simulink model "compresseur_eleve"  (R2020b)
settings: Solver=VariableStepAuto  StartTime=0.0  StopTime=1  RelTol=1e-3
PreLoadFcn:
  | compresseur_7_DataFile
model workspace: external: MATLAB File (data not in the file)
undefined symbols (not defined in the file or in its folder): deg, kg, m, mm, N, s, smiData, X, Y, Z
libraries: sm_lib x91, fl_lib x8, nesl_utility x5, ee_lib x1
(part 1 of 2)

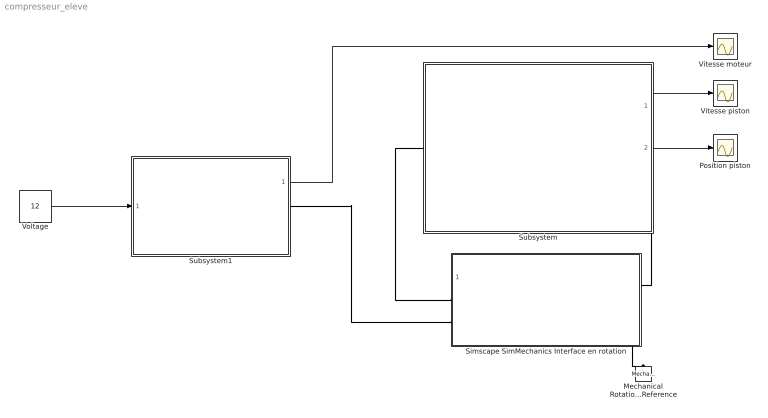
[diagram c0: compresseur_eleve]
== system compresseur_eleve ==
  Mechanical Rotational Reference : fl_lib/Mechanical/Rotational Elements/Mechanical Rotational Reference
  Position piston : Scope
  Simscape SimMechanics Interface en rotation : Subsystem
  Subsystem : Subsystem
  Subsystem1 : Subsystem
  Vitesse moteur : Scope
  Vitesse piston : Scope
  Voltage : Constant  Value=12  VectorParams1D=off  SampleTime=-1
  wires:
  Subsystem/1(output) -> Vitesse piston/1
  Subsystem/2(output1) -> Position piston/1
  Voltage/1 -> Subsystem1/1(input0)
  Subsystem1/1(vitesse de rotation du moteur en tr/mn) -> Vitesse moteur/1
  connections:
  Simscape SimMechanics Interface en rotation/RConn2 -- Mechanical Rotational Reference/LConn1
  Simscape SimMechanics Interface en rotation/LConn1 -- Subsystem/LConn1
  Simscape SimMechanics Interface en rotation/RConn1 -- Subsystem/RConn1
  Simscape SimMechanics Interface en rotation/LConn2 -- Subsystem1/RConn1

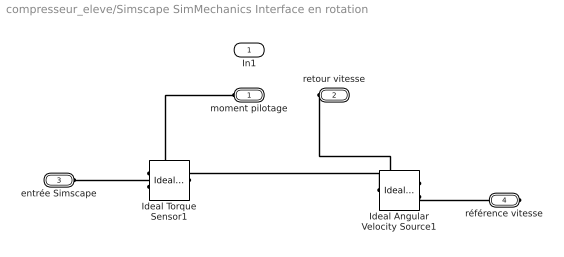
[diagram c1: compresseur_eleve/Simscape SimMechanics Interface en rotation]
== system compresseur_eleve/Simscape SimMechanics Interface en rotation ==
  In1 : Inport
  Ideal Angular Velocity Source1 : fl_lib/Mechanical/Mechanical Sources/Ideal Angular Velocity Source
  Ideal Torque Sensor1 : fl_lib/Mechanical/Mechanical Sensors/Ideal Torque Sensor
  moment pilotage : PMIOPort  Side=Left
  retour vitesse : PMIOPort  Port=2  Side=Right
  entrée Simscape : PMIOPort  Port=3  Side=Left
  référence vitesse : PMIOPort  Port=4  Side=Right
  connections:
  Ideal Angular Velocity Source1/RConn2 -- référence vitesse/RConn1
  Ideal Torque Sensor1/RConn2 -- moment pilotage/RConn1
  Ideal Angular Velocity Source1/LConn1 -- Ideal Torque Sensor1/RConn1
  Ideal Torque Sensor1/LConn1 -- entrée Simscape/RConn1
  retour vitesse/RConn1 -- Ideal Angular Velocity Source1/RConn1

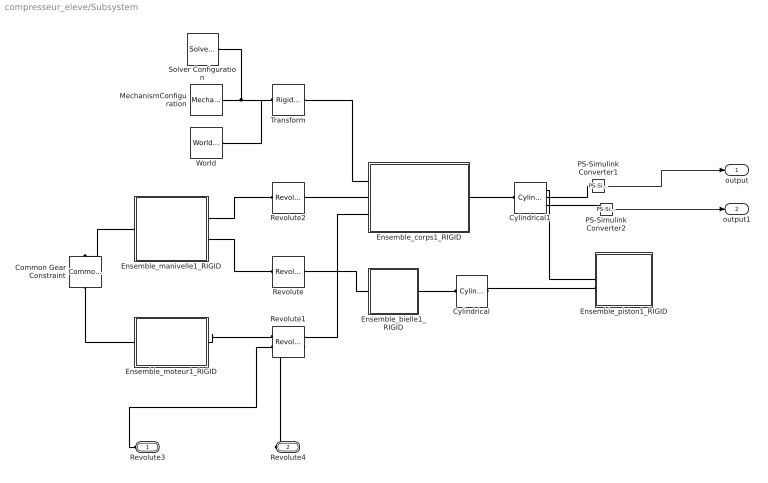
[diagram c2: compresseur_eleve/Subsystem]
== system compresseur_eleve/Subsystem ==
  Common Gear Constraint : sm_lib/Gears and Couplings/Gears/Common Gear Constraint  GearType=External  SpecificationType=CenterDistanceRatio  CenterDistance=22.5  CenterDistanceUnits=mm  GearRatio=3  BaseGearRadius=10.0  BaseGearRadiusUnits=cm  FollGearRadius=10.0  FollGearRadiusUnits=cm  AssemblyGearRotation=Free
  Cylindrical : sm_lib/Joints/Cylindrical Joint  JointMode=Normal  SenseConstraintForce=off  SenseConstraintForceX=off  SenseConstraintForceY=off  SenseConstraintForceZ=off  SenseConstraintTorque=off  SenseConstraintTorqueX=off  SenseConstraintTorqueY=off  SenseConstraintTorqueZ=off  SenseTotalForce=off  SenseTotalForceX=off  SenseTotalForceY=off  SenseTotalForceZ=off  SenseTotalTorque=off  SenseTotalTorqueX=off  SenseTotalTorqueY=off  SenseTotalTorqueZ=off  CompositeWrenchDir=FollowerOnBase  CompositeWrenchFrame=BaseFrame  PzEquilibriumPosition=0  PzEquilibriumPositionUnits=m  PzSpringStiffness=0  PzSpringStiffnessUnits=N/m  PzDampingCoefficient=0  PzDampingCoefficientUnits=N/(m/s)  PzTorqueActuationMode=NoTorque  PzMotionActuationMode=ComputedMotion  PzSensePosition=off  PzSenseVelocity=off  PzSenseAcceleration=off  PzSenseTorqueForce=off  PzSenseLowerLimitTorqueForce=off  PzSenseUpperLimitTorqueForce=off  PzLowerLimitSpecify=off  PzLowerLimitBound=-1  PzLowerLimitBoundUnits=m  PzLowerLimitStiffness=1e6  PzLowerLimitStiffnessUnits=N/m  PzLowerLimitDamping=1e3  PzLowerLimitDampingUnits=N/(m/s)  PzLowerLimitTransitionRegionWidth=1e-4  PzLowerLimitTransitionRegionWidthUnits=m  PzUpperLimitSpecify=off  PzUpperLimitBound=1  PzUpperLimitBoundUnits=m  PzUpperLimitStiffness=1e6  PzUpperLimitStiffnessUnits=N/m  PzUpperLimitDamping=1e3  PzUpperLimitDampingUnits=N/(m/s)  PzUpperLimitTransitionRegionWidth=1e-4  PzUpperLimitTransitionRegionWidthUnits=m  PzPositionTargetSpecify=off  PzPositionTargetPriority=High  PzPositionTargetValue=0  PzPositionTargetValueUnits=m  PzVelocityTargetSpecify=off  PzVelocityTargetPriority=High  PzVelocityTargetValue=0  PzVelocityTargetValueUnits=m/s  RzEquilibriumPosition=0  RzEquilibriumPositionUnits=deg  RzSpringStiffness=0  RzSpringStiffnessUnits=N*m/deg  RzDampingCoefficient=0  RzDampingCoefficientUnits=N*m/(deg/s)  RzTorqueActuationMode=NoTorque  RzMotionActuationMode=ComputedMotion  RzSensePosition=off  RzSenseVelocity=off  RzSenseAcceleration=off  RzSenseTorqueForce=off  RzSenseLowerLimitTorqueForce=off  RzSenseUpperLimitTorqueForce=off  RzLowerLimitSpecify=off  RzLowerLimitBound=-90  RzLowerLimitBoundUnits=deg  RzLowerLimitStiffness=1e4  RzLowerLimitStiffnessUnits=N*m/deg  RzLowerLimitDamping=10  RzLowerLimitDampingUnits=N*m/(deg/s)  RzLowerLimitTransitionRegionWidth=0.1  RzLowerLimitTransitionRegionWidthUnits=deg  RzUpperLimitSpecify=off  RzUpperLimitBound=90  RzUpperLimitBoundUnits=deg  RzUpperLimitStiffness=1e4  RzUpperLimitStiffnessUnits=N*m/deg  RzUpperLimitDamping=10  RzUpperLimitDampingUnits=N*m/(deg/s)  RzUpperLimitTransitionRegionWidth=0.1  RzUpperLimitTransitionRegionWidthUnits=deg  RzPositionTargetSpecify=off  RzPositionTargetPriority=High  RzPositionTargetValue=0  RzPositionTargetValueUnits=deg  RzVelocityTargetSpecify=off  RzVelocityTargetPriority=High  RzVelocityTargetValue=0  RzVelocityTargetValueUnits=deg/s
  Cylindrical1 : sm_lib/Joints/Cylindrical Joint  JointMode=Normal  SenseConstraintForce=off  SenseConstraintForceX=off  SenseConstraintForceY=off  SenseConstraintForceZ=off  SenseConstraintTorque=off  SenseConstraintTorqueX=off  SenseConstraintTorqueY=off  SenseConstraintTorqueZ=off  SenseTotalForce=off  SenseTotalForceX=off  SenseTotalForceY=off  SenseTotalForceZ=off  SenseTotalTorque=off  SenseTotalTorqueX=off  SenseTotalTorqueY=off  SenseTotalTorqueZ=off  CompositeWrenchDir=FollowerOnBase  CompositeWrenchFrame=BaseFrame  PzEquilibriumPosition=0  PzEquilibriumPositionUnits=m  PzSpringStiffness=0  PzSpringStiffnessUnits=N/m  PzDampingCoefficient=0  PzDampingCoefficientUnits=N/(m/s)  PzTorqueActuationMode=NoTorque  PzMotionActuationMode=ComputedMotion  PzSensePosition=on  PzSenseVelocity=on  PzSenseAcceleration=off  PzSenseTorqueForce=off  PzSenseLowerLimitTorqueForce=off  PzSenseUpperLimitTorqueForce=off  PzLowerLimitSpecify=off  PzLowerLimitBound=-1  PzLowerLimitBoundUnits=m  PzLowerLimitStiffness=1e6  PzLowerLimitStiffnessUnits=N/m  PzLowerLimitDamping=1e3  PzLowerLimitDampingUnits=N/(m/s)  PzLowerLimitTransitionRegionWidth=1e-4  PzLowerLimitTransitionRegionWidthUnits=m  PzUpperLimitSpecify=off  PzUpperLimitBound=1  PzUpperLimitBoundUnits=m  PzUpperLimitStiffness=1e6  PzUpperLimitStiffnessUnits=N/m  PzUpperLimitDamping=1e3  PzUpperLimitDampingUnits=N/(m/s)  PzUpperLimitTransitionRegionWidth=1e-4  PzUpperLimitTransitionRegionWidthUnits=m  PzPositionTargetSpecify=on  PzPositionTargetPriority=Low  PzPositionTargetValue=smiData.CylindricalJoint(2).Pz.Pos  PzPositionTargetValueUnits=mm  PzVelocityTargetSpecify=off  PzVelocityTargetPriority=High  PzVelocityTargetValue=0  PzVelocityTargetValueUnits=m/s  RzEquilibriumPosition=0  RzEquilibriumPositionUnits=deg  RzSpringStiffness=0  RzSpringStiffnessUnits=N*m/deg  RzDampingCoefficient=0  RzDampingCoefficientUnits=N*m/(deg/s)  RzTorqueActuationMode=NoTorque  RzMotionActuationMode=ComputedMotion  RzSensePosition=off  RzSenseVelocity=off  RzSenseAcceleration=off  RzSenseTorqueForce=off  RzSenseLowerLimitTorqueForce=off  RzSenseUpperLimitTorqueForce=off  RzLowerLimitSpecify=off  RzLowerLimitBound=-90  RzLowerLimitBoundUnits=deg  RzLowerLimitStiffness=1e4  RzLowerLimitStiffnessUnits=N*m/deg  RzLowerLimitDamping=10  RzLowerLimitDampingUnits=N*m/(deg/s)  RzLowerLimitTransitionRegionWidth=0.1  RzLowerLimitTransitionRegionWidthUnits=deg  RzUpperLimitSpecify=off  RzUpperLimitBound=90  RzUpperLimitBoundUnits=deg  RzUpperLimitStiffness=1e4  RzUpperLimitStiffnessUnits=N*m/deg  RzUpperLimitDamping=10  RzUpperLimitDampingUnits=N*m/(deg/s)  RzUpperLimitTransitionRegionWidth=0.1  RzUpperLimitTransitionRegionWidthUnits=deg  RzPositionTargetSpecify=on  RzPositionTargetPriority=Low  RzPositionTargetValue=smiData.CylindricalJoint(2).Rz.Pos  RzPositionTargetValueUnits=deg  RzVelocityTargetSpecify=off  RzVelocityTargetPriority=High  RzVelocityTargetValue=0  RzVelocityTargetValueUnits=deg/s
  Ensemble_bielle1_RIGID : Subsystem
  Ensemble_corps1_RIGID : Subsystem
  Ensemble_manivelle1_RIGID : Subsystem
  Ensemble_moteur1_RIGID : Subsystem
  Ensemble_piston1_RIGID : Subsystem
  MechanismConfiguration : sm_lib/Utilities/Mechanism Configuration  UniformGravity=Constant  GravityVector=[0 -9.80665 0]  GravityVectorUnits=m/s^2  GravityUnits=m/s^2  LinearizationDelta=0.001  JointModeTransitionNonlinearIterations=2
  PS-Simulink Converter1 : nesl_utility/PS-Simulink Converter  PhysicalDomain=network_engine_domain  SubClassName=ps_output  LeftPortType=input  RightPortType=output  PseudoPeriodic=off  Frequencies=[]  Unit=inherit  AffineConversion=off
  PS-Simulink Converter2 : nesl_utility/PS-Simulink Converter  PhysicalDomain=network_engine_domain  SubClassName=ps_output  LeftPortType=input  RightPortType=output  PseudoPeriodic=off  Frequencies=[]  Unit=inherit  AffineConversion=off
  Revolute : sm_lib/Joints/Revolute Joint  JointMode=Normal  SenseConstraintForce=off  SenseConstraintForceX=off  SenseConstraintForceY=off  SenseConstraintForceZ=off  SenseConstraintTorque=off  SenseConstraintTorqueX=off  SenseConstraintTorqueY=off  SenseConstraintTorqueZ=off  SenseTotalForce=off  SenseTotalForceX=off  SenseTotalForceY=off  SenseTotalForceZ=off  SenseTotalTorque=off  SenseTotalTorqueX=off  SenseTotalTorqueY=off  SenseTotalTorqueZ=off  CompositeWrenchDir=FollowerOnBase  CompositeWrenchFrame=BaseFrame  EquilibriumPosition=0  EquilibriumPositionUnits=deg  SpringStiffness=0  SpringStiffnessUnits=N*m/deg  DampingCoefficient=0  DampingCoefficientUnits=N*m/(deg/s)  TorqueActuationMode=NoTorque  MotionActuationMode=ComputedMotion  SensePosition=off  SenseVelocity=off  SenseAcceleration=off  SenseTorqueForce=off  SenseLowerLimitTorqueForce=off  SenseUpperLimitTorqueForce=off  LowerLimitSpecify=off  LowerLimitBound=-90  LowerLimitBoundUnits=deg  LowerLimitStiffness=1e4  LowerLimitStiffnessUnits=N*m/deg  LowerLimitDamping=10  LowerLimitDampingUnits=N*m/(deg/s)  LowerLimitTransitionRegionWidth=0.1  LowerLimitTransitionRegionWidthUnits=deg  UpperLimitSpecify=off  UpperLimitBound=90  UpperLimitBoundUnits=deg  UpperLimitStiffness=1e4  UpperLimitStiffnessUnits=N*m/deg  UpperLimitDamping=10  UpperLimitDampingUnits=N*m/(deg/s)  UpperLimitTransitionRegionWidth=0.1  UpperLimitTransitionRegionWidthUnits=deg  PositionTargetSpecify=on  PositionTargetPriority=Low  PositionTargetValue=smiData.RevoluteJoint(1).Rz.Pos  PositionTargetValueUnits=deg  VelocityTargetSpecify=off  VelocityTargetPriority=High  VelocityTargetValue=0  VelocityTargetValueUnits=deg/s
  Revolute1 : sm_lib/Joints/Revolute Joint  JointMode=Normal  SenseConstraintForce=off  SenseConstraintForceX=off  SenseConstraintForceY=off  SenseConstraintForceZ=off  SenseConstraintTorque=off  SenseConstraintTorqueX=off  SenseConstraintTorqueY=off  SenseConstraintTorqueZ=off  SenseTotalForce=off  SenseTotalForceX=off  SenseTotalForceY=off  SenseTotalForceZ=off  SenseTotalTorque=off  SenseTotalTorqueX=off  SenseTotalTorqueY=off  SenseTotalTorqueZ=off  CompositeWrenchDir=FollowerOnBase  CompositeWrenchFrame=BaseFrame  EquilibriumPosition=0  EquilibriumPositionUnits=deg  SpringStiffness=0  SpringStiffnessUnits=N*m/deg  DampingCoefficient=0  DampingCoefficientUnits=N*m/(deg/s)  TorqueActuationMode=InputTorque  MotionActuationMode=ComputedMotion  SensePosition=off  SenseVelocity=on  SenseAcceleration=off  SenseTorqueForce=off  SenseLowerLimitTorqueForce=off  SenseUpperLimitTorqueForce=off  LowerLimitSpecify=off  LowerLimitBound=-90  LowerLimitBoundUnits=deg  LowerLimitStiffness=1e4  LowerLimitStiffnessUnits=N*m/deg  LowerLimitDamping=10  LowerLimitDampingUnits=N*m/(deg/s)  LowerLimitTransitionRegionWidth=0.1  LowerLimitTransitionRegionWidthUnits=deg  UpperLimitSpecify=off  UpperLimitBound=90  UpperLimitBoundUnits=deg  UpperLimitStiffness=1e4  UpperLimitStiffnessUnits=N*m/deg  UpperLimitDamping=10  UpperLimitDampingUnits=N*m/(deg/s)  UpperLimitTransitionRegionWidth=0.1  UpperLimitTransitionRegionWidthUnits=deg  PositionTargetSpecify=on  PositionTargetPriority=Low  PositionTargetValue=smiData.RevoluteJoint(2).Rz.Pos  PositionTargetValueUnits=deg  VelocityTargetSpecify=off  VelocityTargetPriority=High  VelocityTargetValue=0  VelocityTargetValueUnits=deg/s
  Revolute2 : sm_lib/Joints/Revolute Joint  JointMode=Normal  SenseConstraintForce=off  SenseConstraintForceX=off  SenseConstraintForceY=off  SenseConstraintForceZ=off  SenseConstraintTorque=off  SenseConstraintTorqueX=off  SenseConstraintTorqueY=off  SenseConstraintTorqueZ=off  SenseTotalForce=off  SenseTotalForceX=off  SenseTotalForceY=off  SenseTotalForceZ=off  SenseTotalTorque=off  SenseTotalTorqueX=off  SenseTotalTorqueY=off  SenseTotalTorqueZ=off  CompositeWrenchDir=FollowerOnBase  CompositeWrenchFrame=BaseFrame  EquilibriumPosition=0  EquilibriumPositionUnits=deg  SpringStiffness=0  SpringStiffnessUnits=N*m/deg  DampingCoefficient=0  DampingCoefficientUnits=N*m/(deg/s)  TorqueActuationMode=NoTorque  MotionActuationMode=ComputedMotion  SensePosition=off  SenseVelocity=off  SenseAcceleration=off  SenseTorqueForce=off  SenseLowerLimitTorqueForce=off  SenseUpperLimitTorqueForce=off  LowerLimitSpecify=off  LowerLimitBound=-90  LowerLimitBoundUnits=deg  LowerLimitStiffness=1e4  LowerLimitStiffnessUnits=N*m/deg  LowerLimitDamping=10  LowerLimitDampingUnits=N*m/(deg/s)  LowerLimitTransitionRegionWidth=0.1  LowerLimitTransitionRegionWidthUnits=deg  UpperLimitSpecify=off  UpperLimitBound=90  UpperLimitBoundUnits=deg  UpperLimitStiffness=1e4  UpperLimitStiffnessUnits=N*m/deg  UpperLimitDamping=10  UpperLimitDampingUnits=N*m/(deg/s)  UpperLimitTransitionRegionWidth=0.1  UpperLimitTransitionRegionWidthUnits=deg  PositionTargetSpecify=on  PositionTargetPriority=Low  PositionTargetValue=smiData.RevoluteJoint(3).Rz.Pos  PositionTargetValueUnits=deg  VelocityTargetSpecify=off  VelocityTargetPriority=High  VelocityTargetValue=0  VelocityTargetValueUnits=deg/s
  Solver Configuration : nesl_utility/Solver Configuration  PhysicalDomain=network_engine_domain  SubClassName=solver  LeftPortType=input  RightPortType=generic  Tones=[]  Harmonics=[]  SimulateNoise=off  Profile=off  UseLocalSampling=off  EnableSwitchedLinearOptims=on  FrequencyDomain=off  UseCCode=off  RelTol=0.001  AbsTol=1e-06  MinStep=1e-09  ToWorkspace=off  RevertToSquareIcSolve=off  NumHomotopyIterations=100  PhasorMode=off  PhasorModeNumHarmonics=1  DoDC=off  ResidualTolerance=1e-09  UseLocalSolver=off  LocalSolverChoice=NE_BACKWARD_EULER_ADVANCER  LocalSolverSampleTime=0.001  DoFixedCost=off  MaxNonlinIter=3  MaxModeIter=2  ComputeImpulses=off  ImpulseIterations=2  LinearAlgebra=auto  EquationFormulation=NE_TIME_EF  DelaysMemoryBudget=1024  AutomaticFiltering=on  FilteringTimeConstant=0.001  PartitionStorageMethod=AS_NEEDED  PartitionMemoryBudget=1024  PartitionMethod=ROBUST
  Transform : sm_lib/Frames and Transforms/Rigid Transform  TranslationMethod=Cartesian  TranslationStandardOffset=0  TranslationLengthUnit=mm  TranslationStandardAxis=+Z  TranslationCartesianOffset=smiData.RigidTransform(33).translation  TranslationROffset=0  TranslationROffsetUnits=m  TranslationZOffset=0  TranslationZOffsetUnits=m  TranslationThetaOffset=0  TranslationThetaOffsetUnits=deg  RotationMethod=ArbitraryAxis  RotationAngleUnits=rad  RotationStandardAxis=+Z  RotationAngle=smiData.RigidTransform(33).angle  RotationArbitraryAxis=smiData.RigidTransform(33).axis  FollAlignAxisA=+X  BaseAlignAxisA=+Y  FollAlignAxisB=+Y  BaseAlignAxisB=+Z  RotationSequenceAxes=FollowerAxes  RotationSequence=XYX  RotationSequenceAngles=[0 0 0]  RotationSequenceAnglesUnits=deg  RotationMatrix=[1 0 0; 0 1 0; 0 0 1]
  World : sm_lib/Frames and Transforms/World Frame
  Revolute3 : PMIOPort  Side=Left
  Revolute4 : PMIOPort  Port=2  Side=Right
  output : Outport
  output1 : Outport  Port=2
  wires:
  PS-Simulink Converter2/1 -> output1/1
  PS-Simulink Converter1/1 -> output/1
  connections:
  Transform/LConn1 -- MechanismConfiguration/RConn1 -- Solver Configuration/RConn1 -- World/RConn1
  Cylindrical1/LConn1 -- Ensemble_corps1_RIGID/RConn1
  Ensemble_corps1_RIGID/LConn1 -- Transform/RConn1
  PS-Simulink Converter1/LConn1 -- Cylindrical1/RConn2
  Ensemble_corps1_RIGID/LConn3 -- Revolute1/RConn1
  Ensemble_manivelle1_RIGID/RConn1 -- Revolute2/LConn1
  PS-Simulink Converter2/LConn1 -- Cylindrical1/RConn3
  Revolute3/RConn1 -- Revolute1/LConn2
  Common Gear Constraint/LConn1 -- Ensemble_moteur1_RIGID/LConn1
  Ensemble_manivelle1_RIGID/RConn2 -- Revolute/LConn1
  Cylindrical/RConn1 -- Ensemble_piston1_RIGID/LConn2
  Ensemble_corps1_RIGID/LConn2 -- Revolute2/RConn1
  Cylindrical1/RConn1 -- Ensemble_piston1_RIGID/LConn1
  Cylindrical/LConn1 -- Ensemble_bielle1_RIGID/RConn1
  Ensemble_moteur1_RIGID/RConn1 -- Revolute1/LConn1
  Ensemble_manivelle1_RIGID/LConn1 -- Common Gear Constraint/RConn1
  Ensemble_bielle1_RIGID/LConn1 -- Revolute/RConn1
  Revolute4/RConn1 -- Revolute1/RConn2

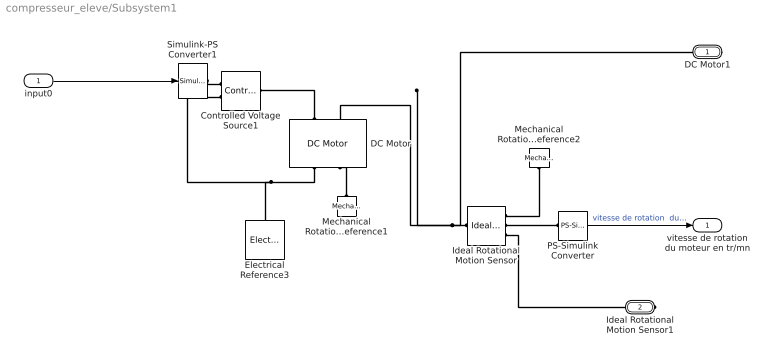
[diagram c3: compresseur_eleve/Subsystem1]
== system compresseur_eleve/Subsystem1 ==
  input0 : Inport
  Controlled Voltage Source1 : fl_lib/Electrical/Electrical Sources/Controlled Voltage Source
  DC Motor : ee_lib/Electromechanical/Brushed Motors/DC Motor  field_option=ee.enum.field_option.pm  Rf=100 Ohm  Lf=1 H  Laf=0.15 H  If0=0 A  parameterization=1  Ra=3.9 Ohm  La=0.1 mH  emf_or_torque=2  Kv=7.2e-6 V/rpm  Ki=1e-2 N*m/A  T_stall=2.4e-4 N*m  w_max=1.91e+4 rpm  w_rated=1.5e+4 rpm  P_rated=0.08 W  V_rated=1.5 V  J=80 g*cm^2  lam_param=1  lam=0 N*m/(rad/s)  i_noload=0 A  V_i_noload=1.5 V  speed0=0 rpm  enable_fault_armature=ee.enum.faults.faultEnable.no  rev_faulted=1 / 3  G_faulted_armature=1e-5 S  fault_trigger_armature=ee.enum.faults.faultTrigger.temporal  t_fault_armature=1 s  max_permissible_current_armature=inf A  t_fail_on_current_armature=1 s  enable_fault_field=ee.enum.faults.faultEnable.no  G_faulted_field=1e-5 S  fault_trigger_field=ee.enum.faults.faultTrigger.temporal  t_fault_field=1 s  max_permissible_current_field=inf A  t_fail_on_current_field=1 s  fault_action=ee.enum.faults.faultAction.none  alpha=3.93e-3 1/K  Tmeas=25 degC  thermal_mass=100 J/K  initial_temperature=25 degC
  Electrical Reference3 : fl_lib/Electrical/Electrical Elements/Electrical Reference
  Ideal Rotational Motion Sensor : fl_lib/Mechanical/Mechanical Sensors/Ideal Rotational Motion Sensor  wrap_angle=simscape.enum.onoff.off  offset=0 rad
  Mechanical Rotational Reference1 : fl_lib/Mechanical/Rotational Elements/Mechanical Rotational Reference
  Mechanical Rotational Reference2 : fl_lib/Mechanical/Rotational Elements/Mechanical Rotational Reference
  PS-Simulink Converter : nesl_utility/PS-Simulink Converter  PhysicalDomain=network_engine_domain  SubClassName=ps_output  LeftPortType=input  RightPortType=output  PseudoPeriodic=off  Frequencies=[]  Unit=rpm  AffineConversion=off
  Simulink-PS Converter1 : nesl_utility/Simulink-PS Converter  PhysicalDomain=network_engine_domain  SubClassName=ps_input  LeftPortType=input  RightPortType=output  PseudoPeriodic=off  Frequencies=[]  NoiseDistribution=none  NoiseParameters=[]  Unit=V  AffineConversion=off  FilteringAndDerivatives=zero  SimscapeFilterOrder=1  InputFilterTimeConstant=0.001  UdotUserProvided=1
  DC Motor1 : PMIOPort  Side=Right
  Ideal Rotational Motion Sensor1 : PMIOPort  Port=2  Side=Right
  vitesse de rotation du moteur en tr/mn : Outport
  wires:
  input0/1 -> Simulink-PS Converter1/1
  PS-Simulink Converter/1 -> vitesse de rotation du moteur en tr/mn/1  "vitesse de rotation  du moteur en tr/mn"
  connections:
  Mechanical Rotational Reference2/LConn1 -- Ideal Rotational Motion Sensor/RConn1
  DC Motor/RConn1 -- Controlled Voltage Source1/RConn2 -- Electrical Reference3/LConn1
  Ideal Rotational Motion Sensor/RConn2 -- PS-Simulink Converter/LConn1
  Ideal Rotational Motion Sensor/LConn1 -- DC Motor1/RConn1 -- DC Motor/LConn2
  DC Motor/LConn1 -- Controlled Voltage Source1/LConn1
  Ideal Rotational Motion Sensor/RConn3 -- Ideal Rotational Motion Sensor1/RConn1
  Simulink-PS Converter1/RConn1 -- Controlled Voltage Source1/RConn1
  Mechanical Rotational Reference1/LConn1 -- DC Motor/RConn2

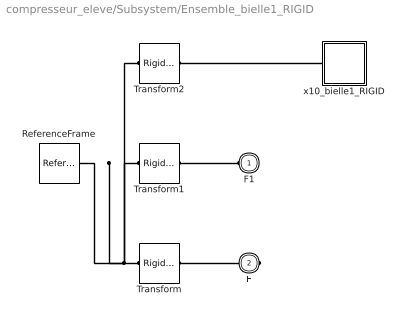
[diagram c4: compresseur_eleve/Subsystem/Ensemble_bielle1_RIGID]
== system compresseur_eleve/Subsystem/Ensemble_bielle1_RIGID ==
  ReferenceFrame : sm_lib/Frames and Transforms/Reference Frame
  Transform : sm_lib/Frames and Transforms/Rigid Transform  TranslationMethod=Cartesian  TranslationStandardOffset=0  TranslationLengthUnit=mm  TranslationStandardAxis=+Z  TranslationCartesianOffset=smiData.RigidTransform(1).translation  TranslationROffset=0  TranslationROffsetUnits=m  TranslationZOffset=0  TranslationZOffsetUnits=m  TranslationThetaOffset=0  TranslationThetaOffsetUnits=deg  RotationMethod=ArbitraryAxis  RotationAngleUnits=rad  RotationStandardAxis=+Z  RotationAngle=smiData.RigidTransform(1).angle  RotationArbitraryAxis=smiData.RigidTransform(1).axis  FollAlignAxisA=+X  BaseAlignAxisA=+Y  FollAlignAxisB=+Y  BaseAlignAxisB=+Z  RotationSequenceAxes=FollowerAxes  RotationSequence=XYX  RotationSequenceAngles=[0 0 0]  RotationSequenceAnglesUnits=deg  RotationMatrix=[1 0 0; 0 1 0; 0 0 1]
  Transform1 : sm_lib/Frames and Transforms/Rigid Transform  TranslationMethod=Cartesian  TranslationStandardOffset=0  TranslationLengthUnit=mm  TranslationStandardAxis=+Z  TranslationCartesianOffset=smiData.RigidTransform(4).translation  TranslationROffset=0  TranslationROffsetUnits=m  TranslationZOffset=0  TranslationZOffsetUnits=m  TranslationThetaOffset=0  TranslationThetaOffsetUnits=deg  RotationMethod=ArbitraryAxis  RotationAngleUnits=rad  RotationStandardAxis=+Z  RotationAngle=smiData.RigidTransform(4).angle  RotationArbitraryAxis=smiData.RigidTransform(4).axis  FollAlignAxisA=+X  BaseAlignAxisA=+Y  FollAlignAxisB=+Y  BaseAlignAxisB=+Z  RotationSequenceAxes=FollowerAxes  RotationSequence=XYX  RotationSequenceAngles=[0 0 0]  RotationSequenceAnglesUnits=deg  RotationMatrix=[1 0 0; 0 1 0; 0 0 1]
  Transform2 : sm_lib/Frames and Transforms/Rigid Transform  TranslationMethod=Cartesian  TranslationStandardOffset=0  TranslationLengthUnit=mm  TranslationStandardAxis=+Z  TranslationCartesianOffset=smiData.RigidTransform(20).translation  TranslationROffset=0  TranslationROffsetUnits=m  TranslationZOffset=0  TranslationZOffsetUnits=m  TranslationThetaOffset=0  TranslationThetaOffsetUnits=deg  RotationMethod=ArbitraryAxis  RotationAngleUnits=rad  RotationStandardAxis=+Z  RotationAngle=smiData.RigidTransform(20).angle  RotationArbitraryAxis=smiData.RigidTransform(20).axis  FollAlignAxisA=+X  BaseAlignAxisA=+Y  FollAlignAxisB=+Y  BaseAlignAxisB=+Z  RotationSequenceAxes=FollowerAxes  RotationSequence=XYX  RotationSequenceAngles=[0 0 0]  RotationSequenceAnglesUnits=deg  RotationMatrix=[1 0 0; 0 1 0; 0 0 1]
  x10_bielle1_RIGID : Subsystem
  F1 : PMIOPort  Side=Left
  F : PMIOPort  Port=2  Side=Right
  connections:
  Transform/LConn1 -- ReferenceFrame/RConn1 -- Transform1/LConn1 -- Transform2/LConn1
  Transform/RConn1 -- F/RConn1
  Transform1/RConn1 -- F1/RConn1
  Transform2/RConn1 -- x10_bielle1_RIGID/LConn1

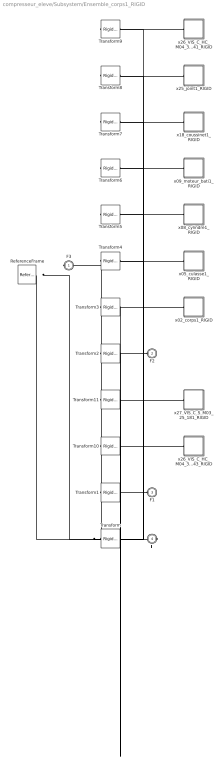
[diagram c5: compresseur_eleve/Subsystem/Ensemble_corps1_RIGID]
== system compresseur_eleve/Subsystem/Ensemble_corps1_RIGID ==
  ReferenceFrame : sm_lib/Frames and Transforms/Reference Frame
  Transform : sm_lib/Frames and Transforms/Rigid Transform  TranslationMethod=Cartesian  TranslationStandardOffset=0  TranslationLengthUnit=mm  TranslationStandardAxis=+Z  TranslationCartesianOffset=smiData.RigidTransform(5).translation  TranslationROffset=0  TranslationROffsetUnits=m  TranslationZOffset=0  TranslationZOffsetUnits=m  TranslationThetaOffset=0  TranslationThetaOffsetUnits=deg  RotationMethod=ArbitraryAxis  RotationAngleUnits=rad  RotationStandardAxis=+Z  RotationAngle=smiData.RigidTransform(5).angle  RotationArbitraryAxis=smiData.RigidTransform(5).axis  FollAlignAxisA=+X  BaseAlignAxisA=+Y  FollAlignAxisB=+Y  BaseAlignAxisB=+Z  RotationSequenceAxes=FollowerAxes  RotationSequence=XYX  RotationSequenceAngles=[0 0 0]  RotationSequenceAnglesUnits=deg  RotationMatrix=[1 0 0; 0 1 0; 0 0 1]
  Transform1 : sm_lib/Frames and Transforms/Rigid Transform  TranslationMethod=Cartesian  TranslationStandardOffset=0  TranslationLengthUnit=mm  TranslationStandardAxis=+Z  TranslationCartesianOffset=smiData.RigidTransform(8).translation  TranslationROffset=0  TranslationROffsetUnits=m  TranslationZOffset=0  TranslationZOffsetUnits=m  TranslationThetaOffset=0  TranslationThetaOffsetUnits=deg  RotationMethod=ArbitraryAxis  RotationAngleUnits=rad  RotationStandardAxis=+Z  RotationAngle=smiData.RigidTransform(8).angle  RotationArbitraryAxis=smiData.RigidTransform(8).axis  FollAlignAxisA=+X  BaseAlignAxisA=+Y  FollAlignAxisB=+Y  BaseAlignAxisB=+Z  RotationSequenceAxes=FollowerAxes  RotationSequence=XYX  RotationSequenceAngles=[0 0 0]  RotationSequenceAnglesUnits=deg  RotationMatrix=[1 0 0; 0 1 0; 0 0 1]
  Transform10 : sm_lib/Frames and Transforms/Rigid Transform  TranslationMethod=Cartesian  TranslationStandardOffset=0  TranslationLengthUnit=mm  TranslationStandardAxis=+Z  TranslationCartesianOffset=smiData.RigidTransform(18).translation  TranslationROffset=0  TranslationROffsetUnits=m  TranslationZOffset=0  TranslationZOffsetUnits=m  TranslationThetaOffset=0  TranslationThetaOffsetUnits=deg  RotationMethod=ArbitraryAxis  RotationAngleUnits=rad  RotationStandardAxis=+Z  RotationAngle=smiData.RigidTransform(18).angle  RotationArbitraryAxis=smiData.RigidTransform(18).axis  FollAlignAxisA=+X  BaseAlignAxisA=+Y  FollAlignAxisB=+Y  BaseAlignAxisB=+Z  RotationSequenceAxes=FollowerAxes  RotationSequence=XYX  RotationSequenceAngles=[0 0 0]  RotationSequenceAnglesUnits=deg  RotationMatrix=[1 0 0; 0 1 0; 0 0 1]
  Transform11 : sm_lib/Frames and Transforms/Rigid Transform  TranslationMethod=Cartesian  TranslationStandardOffset=0  TranslationLengthUnit=mm  TranslationStandardAxis=+Z  TranslationCartesianOffset=smiData.RigidTransform(19).translation  TranslationROffset=0  TranslationROffsetUnits=m  TranslationZOffset=0  TranslationZOffsetUnits=m  TranslationThetaOffset=0  TranslationThetaOffsetUnits=deg  RotationMethod=ArbitraryAxis  RotationAngleUnits=rad  RotationStandardAxis=+Z  RotationAngle=smiData.RigidTransform(19).angle  RotationArbitraryAxis=smiData.RigidTransform(19).axis  FollAlignAxisA=+X  BaseAlignAxisA=+Y  FollAlignAxisB=+Y  BaseAlignAxisB=+Z  RotationSequenceAxes=FollowerAxes  RotationSequence=XYX  RotationSequenceAngles=[0 0 0]  RotationSequenceAnglesUnits=deg  RotationMatrix=[1 0 0; 0 1 0; 0 0 1]
  Transform2 : sm_lib/Frames and Transforms/Rigid Transform  TranslationMethod=Cartesian  TranslationStandardOffset=0  TranslationLengthUnit=mm  TranslationStandardAxis=+Z  TranslationCartesianOffset=smiData.RigidTransform(10).translation  TranslationROffset=0  TranslationROffsetUnits=m  TranslationZOffset=0  TranslationZOffsetUnits=m  TranslationThetaOffset=0  TranslationThetaOffsetUnits=deg  RotationMethod=ArbitraryAxis  RotationAngleUnits=rad  RotationStandardAxis=+Z  RotationAngle=smiData.RigidTransform(10).angle  RotationArbitraryAxis=smiData.RigidTransform(10).axis  FollAlignAxisA=+X  BaseAlignAxisA=+Y  FollAlignAxisB=+Y  BaseAlignAxisB=+Z  RotationSequenceAxes=FollowerAxes  RotationSequence=XYX  RotationSequenceAngles=[0 0 0]  RotationSequenceAnglesUnits=deg  RotationMatrix=[1 0 0; 0 1 0; 0 0 1]
  Transform3 : sm_lib/Frames and Transforms/Rigid Transform  TranslationMethod=Cartesian  TranslationStandardOffset=0  TranslationLengthUnit=mm  TranslationStandardAxis=+Z  TranslationCartesianOffset=smiData.RigidTransform(11).translation  TranslationROffset=0  TranslationROffsetUnits=m  TranslationZOffset=0  TranslationZOffsetUnits=m  TranslationThetaOffset=0  TranslationThetaOffsetUnits=deg  RotationMethod=ArbitraryAxis  RotationAngleUnits=rad  RotationStandardAxis=+Z  RotationAngle=smiData.RigidTransform(11).angle  RotationArbitraryAxis=smiData.RigidTransform(11).axis  FollAlignAxisA=+X  BaseAlignAxisA=+Y  FollAlignAxisB=+Y  BaseAlignAxisB=+Z  RotationSequenceAxes=FollowerAxes  RotationSequence=XYX  RotationSequenceAngles=[0 0 0]  RotationSequenceAnglesUnits=deg  RotationMatrix=[1 0 0; 0 1 0; 0 0 1]
  Transform4 : sm_lib/Frames and Transforms/Rigid Transform  TranslationMethod=Cartesian  TranslationStandardOffset=0  TranslationLengthUnit=mm  TranslationStandardAxis=+Z  TranslationCartesianOffset=smiData.RigidTransform(12).translation  TranslationROffset=0  TranslationROffsetUnits=m  TranslationZOffset=0  TranslationZOffsetUnits=m  TranslationThetaOffset=0  TranslationThetaOffsetUnits=deg  RotationMethod=ArbitraryAxis  RotationAngleUnits=rad  RotationStandardAxis=+Z  RotationAngle=smiData.RigidTransform(12).angle  RotationArbitraryAxis=smiData.RigidTransform(12).axis  FollAlignAxisA=+X  BaseAlignAxisA=+Y  FollAlignAxisB=+Y  BaseAlignAxisB=+Z  RotationSequenceAxes=FollowerAxes  RotationSequence=XYX  RotationSequenceAngles=[0 0 0]  RotationSequenceAnglesUnits=deg  RotationMatrix=[1 0 0; 0 1 0; 0 0 1]
  Transform5 : sm_lib/Frames and Transforms/Rigid Transform  TranslationMethod=Cartesian  TranslationStandardOffset=0  TranslationLengthUnit=mm  TranslationStandardAxis=+Z  TranslationCartesianOffset=smiData.RigidTransform(13).translation  TranslationROffset=0  TranslationROffsetUnits=m  TranslationZOffset=0  TranslationZOffsetUnits=m  TranslationThetaOffset=0  TranslationThetaOffsetUnits=deg  RotationMethod=ArbitraryAxis  RotationAngleUnits=rad  RotationStandardAxis=+Z  RotationAngle=smiData.RigidTransform(13).angle  RotationArbitraryAxis=smiData.RigidTransform(13).axis  FollAlignAxisA=+X  BaseAlignAxisA=+Y  FollAlignAxisB=+Y  BaseAlignAxisB=+Z  RotationSequenceAxes=FollowerAxes  RotationSequence=XYX  RotationSequenceAngles=[0 0 0]  RotationSequenceAnglesUnits=deg  RotationMatrix=[1 0 0; 0 1 0; 0 0 1]
  Transform6 : sm_lib/Frames and Transforms/Rigid Transform  TranslationMethod=Cartesian  TranslationStandardOffset=0  TranslationLengthUnit=mm  TranslationStandardAxis=+Z  TranslationCartesianOffset=smiData.RigidTransform(14).translation  TranslationROffset=0  TranslationROffsetUnits=m  TranslationZOffset=0  TranslationZOffsetUnits=m  TranslationThetaOffset=0  TranslationThetaOffsetUnits=deg  RotationMethod=ArbitraryAxis  RotationAngleUnits=rad  RotationStandardAxis=+Z  RotationAngle=smiData.RigidTransform(14).angle  RotationArbitraryAxis=smiData.RigidTransform(14).axis  FollAlignAxisA=+X  BaseAlignAxisA=+Y  FollAlignAxisB=+Y  BaseAlignAxisB=+Z  RotationSequenceAxes=FollowerAxes  RotationSequence=XYX  RotationSequenceAngles=[0 0 0]  RotationSequenceAnglesUnits=deg  RotationMatrix=[1 0 0; 0 1 0; 0 0 1]
  Transform7 : sm_lib/Frames and Transforms/Rigid Transform  TranslationMethod=Cartesian  TranslationStandardOffset=0  TranslationLengthUnit=mm  TranslationStandardAxis=+Z  TranslationCartesianOffset=smiData.RigidTransform(15).translation  TranslationROffset=0  TranslationROffsetUnits=m  TranslationZOffset=0  TranslationZOffsetUnits=m  TranslationThetaOffset=0  TranslationThetaOffsetUnits=deg  RotationMethod=ArbitraryAxis  RotationAngleUnits=rad  RotationStandardAxis=+Z  RotationAngle=smiData.RigidTransform(15).angle  RotationArbitraryAxis=smiData.RigidTransform(15).axis  FollAlignAxisA=+X  BaseAlignAxisA=+Y  FollAlignAxisB=+Y  BaseAlignAxisB=+Z  RotationSequenceAxes=FollowerAxes  RotationSequence=XYX  RotationSequenceAngles=[0 0 0]  RotationSequenceAnglesUnits=deg  RotationMatrix=[1 0 0; 0 1 0; 0 0 1]
  Transform8 : sm_lib/Frames and Transforms/Rigid Transform  TranslationMethod=Cartesian  TranslationStandardOffset=0  TranslationLengthUnit=mm  TranslationStandardAxis=+Z  TranslationCartesianOffset=smiData.RigidTransform(16).translation  TranslationROffset=0  TranslationROffsetUnits=m  TranslationZOffset=0  TranslationZOffsetUnits=m  TranslationThetaOffset=0  TranslationThetaOffsetUnits=deg  RotationMethod=ArbitraryAxis  RotationAngleUnits=rad  RotationStandardAxis=+Z  RotationAngle=smiData.RigidTransform(16).angle  RotationArbitraryAxis=smiData.RigidTransform(16).axis  FollAlignAxisA=+X  BaseAlignAxisA=+Y  FollAlignAxisB=+Y  BaseAlignAxisB=+Z  RotationSequenceAxes=FollowerAxes  RotationSequence=XYX  RotationSequenceAngles=[0 0 0]  RotationSequenceAnglesUnits=deg  RotationMatrix=[1 0 0; 0 1 0; 0 0 1]
  Transform9 : sm_lib/Frames and Transforms/Rigid Transform  TranslationMethod=Cartesian  TranslationStandardOffset=0  TranslationLengthUnit=mm  TranslationStandardAxis=+Z  TranslationCartesianOffset=smiData.RigidTransform(17).translation  TranslationROffset=0  TranslationROffsetUnits=m  TranslationZOffset=0  TranslationZOffsetUnits=m  TranslationThetaOffset=0  TranslationThetaOffsetUnits=deg  RotationMethod=ArbitraryAxis  RotationAngleUnits=rad  RotationStandardAxis=+Z  RotationAngle=smiData.RigidTransform(17).angle  RotationArbitraryAxis=smiData.RigidTransform(17).axis  FollAlignAxisA=+X  BaseAlignAxisA=+Y  FollAlignAxisB=+Y  BaseAlignAxisB=+Z  RotationSequenceAxes=FollowerAxes  RotationSequence=XYX  RotationSequenceAngles=[0 0 0]  RotationSequenceAnglesUnits=deg  RotationMatrix=[1 0 0; 0 1 0; 0 0 1]
  x02_corps1_RIGID : Subsystem
  x05_culasse1_RIGID : Subsystem
  x08_cylindre1_RIGID : Subsystem
  x09_moteur_bati1_RIGID : Subsystem
  x18_coussinet1_RIGID : Subsystem
  x25_joint1_RIGID : Subsystem
  x26_VIS_C_HC_M04_35_141_RIGID : Subsystem
  x26_VIS_C_HC_M04_35_143_RIGID : Subsystem
  x27_VIS_C_S_M03_25_181_RIGID : Subsystem
  F3 : PMIOPort  Side=Left
  F2 : PMIOPort  Port=2  Side=Left
  F1 : PMIOPort  Port=3  Side=Left
  F : PMIOPort  Port=4  Side=Right
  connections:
  Transform/LConn1 -- ReferenceFrame/RConn1 -- Transform1/LConn1 -- Transform10/LConn1 -- Transform11/LConn1 -- Transform2/LConn1 -- Transform3/LConn1 -- Transform4/LConn1 -- Transform5/LConn1 -- Transform6/LConn1 -- Transform7/LConn1 -- Transform8/LConn1 -- Transform9/LConn1 -- F3/RConn1
  Transform/RConn1 -- F/RConn1
  Transform9/RConn1 -- x26_VIS_C_HC_M04_35_141_RIGID/LConn1
  Transform10/RConn1 -- x26_VIS_C_HC_M04_35_143_RIGID/LConn1
  Transform11/RConn1 -- x27_VIS_C_S_M03_25_181_RIGID/LConn1
  Transform1/RConn1 -- F1/RConn1
  Transform2/RConn1 -- F2/RConn1
  Transform3/RConn1 -- x02_corps1_RIGID/LConn1
  Transform4/RConn1 -- x05_culasse1_RIGID/LConn1
  Transform5/RConn1 -- x08_cylindre1_RIGID/LConn1
  Transform6/RConn1 -- x09_moteur_bati1_RIGID/LConn1
  Transform7/RConn1 -- x18_coussinet1_RIGID/LConn1
  Transform8/RConn1 -- x25_joint1_RIGID/LConn1

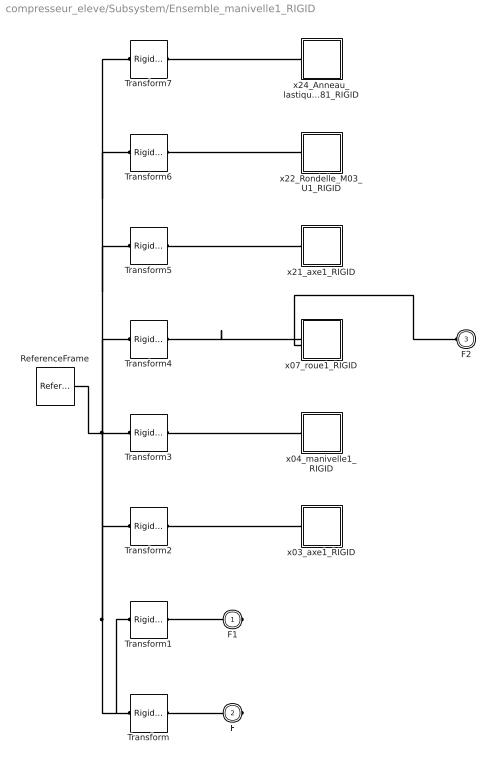
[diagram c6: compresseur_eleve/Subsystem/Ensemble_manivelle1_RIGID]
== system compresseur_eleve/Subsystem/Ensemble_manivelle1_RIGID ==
  ReferenceFrame : sm_lib/Frames and Transforms/Reference Frame
  Transform : sm_lib/Frames and Transforms/Rigid Transform  TranslationMethod=Cartesian  TranslationStandardOffset=0  TranslationLengthUnit=mm  TranslationStandardAxis=+Z  TranslationCartesianOffset=smiData.RigidTransform(3).translation  TranslationROffset=0  TranslationROffsetUnits=m  TranslationZOffset=0  TranslationZOffsetUnits=m  TranslationThetaOffset=0  TranslationThetaOffsetUnits=deg  RotationMethod=ArbitraryAxis  RotationAngleUnits=rad  RotationStandardAxis=+Z  RotationAngle=smiData.RigidTransform(3).angle  RotationArbitraryAxis=smiData.RigidTransform(3).axis  FollAlignAxisA=+X  BaseAlignAxisA=+Y  FollAlignAxisB=+Y  BaseAlignAxisB=+Z  RotationSequenceAxes=FollowerAxes  RotationSequence=XYX  RotationSequenceAngles=[0 0 0]  RotationSequenceAnglesUnits=deg  RotationMatrix=[1 0 0; 0 1 0; 0 0 1]
  Transform1 : sm_lib/Frames and Transforms/Rigid Transform  TranslationMethod=Cartesian  TranslationStandardOffset=0  TranslationLengthUnit=mm  TranslationStandardAxis=+Z  TranslationCartesianOffset=smiData.RigidTransform(9).translation  TranslationROffset=0  TranslationROffsetUnits=m  TranslationZOffset=0  TranslationZOffsetUnits=m  TranslationThetaOffset=0  TranslationThetaOffsetUnits=deg  RotationMethod=ArbitraryAxis  RotationAngleUnits=rad  RotationStandardAxis=+Z  RotationAngle=smiData.RigidTransform(9).angle  RotationArbitraryAxis=smiData.RigidTransform(9).axis  FollAlignAxisA=+X  BaseAlignAxisA=+Y  FollAlignAxisB=+Y  BaseAlignAxisB=+Z  RotationSequenceAxes=FollowerAxes  RotationSequence=XYX  RotationSequenceAngles=[0 0 0]  RotationSequenceAnglesUnits=deg  RotationMatrix=[1 0 0; 0 1 0; 0 0 1]
  Transform2 : sm_lib/Frames and Transforms/Rigid Transform  TranslationMethod=Cartesian  TranslationStandardOffset=0  TranslationLengthUnit=mm  TranslationStandardAxis=+Z  TranslationCartesianOffset=smiData.RigidTransform(25).translation  TranslationROffset=0  TranslationROffsetUnits=m  TranslationZOffset=0  TranslationZOffsetUnits=m  TranslationThetaOffset=0  TranslationThetaOffsetUnits=deg  RotationMethod=ArbitraryAxis  RotationAngleUnits=rad  RotationStandardAxis=+Z  RotationAngle=smiData.RigidTransform(25).angle  RotationArbitraryAxis=smiData.RigidTransform(25).axis  FollAlignAxisA=+X  BaseAlignAxisA=+Y  FollAlignAxisB=+Y  BaseAlignAxisB=+Z  RotationSequenceAxes=FollowerAxes  RotationSequence=XYX  RotationSequenceAngles=[0 0 0]  RotationSequenceAnglesUnits=deg  RotationMatrix=[1 0 0; 0 1 0; 0 0 1]
  Transform3 : sm_lib/Frames and Transforms/Rigid Transform  TranslationMethod=Cartesian  TranslationStandardOffset=0  TranslationLengthUnit=mm  TranslationStandardAxis=+Z  TranslationCartesianOffset=smiData.RigidTransform(26).translation  TranslationROffset=0  TranslationROffsetUnits=m  TranslationZOffset=0  TranslationZOffsetUnits=m  TranslationThetaOffset=0  TranslationThetaOffsetUnits=deg  RotationMethod=ArbitraryAxis  RotationAngleUnits=rad  RotationStandardAxis=+Z  RotationAngle=smiData.RigidTransform(26).angle  RotationArbitraryAxis=smiData.RigidTransform(26).axis  FollAlignAxisA=+X  BaseAlignAxisA=+Y  FollAlignAxisB=+Y  BaseAlignAxisB=+Z  RotationSequenceAxes=FollowerAxes  RotationSequence=XYX  RotationSequenceAngles=[0 0 0]  RotationSequenceAnglesUnits=deg  RotationMatrix=[1 0 0; 0 1 0; 0 0 1]
  Transform4 : sm_lib/Frames and Transforms/Rigid Transform  TranslationMethod=Cartesian  TranslationStandardOffset=0  TranslationLengthUnit=mm  TranslationStandardAxis=+Z  TranslationCartesianOffset=smiData.RigidTransform(27).translation  TranslationROffset=0  TranslationROffsetUnits=m  TranslationZOffset=0  TranslationZOffsetUnits=m  TranslationThetaOffset=0  TranslationThetaOffsetUnits=deg  RotationMethod=ArbitraryAxis  RotationAngleUnits=rad  RotationStandardAxis=+Z  RotationAngle=smiData.RigidTransform(27).angle  RotationArbitraryAxis=smiData.RigidTransform(27).axis  FollAlignAxisA=+X  BaseAlignAxisA=+Y  FollAlignAxisB=+Y  BaseAlignAxisB=+Z  RotationSequenceAxes=FollowerAxes  RotationSequence=XYX  RotationSequenceAngles=[0 0 0]  RotationSequenceAnglesUnits=deg  RotationMatrix=[1 0 0; 0 1 0; 0 0 1]
  Transform5 : sm_lib/Frames and Transforms/Rigid Transform  TranslationMethod=Cartesian  TranslationStandardOffset=0  TranslationLengthUnit=mm  TranslationStandardAxis=+Z  TranslationCartesianOffset=smiData.RigidTransform(28).translation  TranslationROffset=0  TranslationROffsetUnits=m  TranslationZOffset=0  TranslationZOffsetUnits=m  TranslationThetaOffset=0  TranslationThetaOffsetUnits=deg  RotationMethod=ArbitraryAxis  RotationAngleUnits=rad  RotationStandardAxis=+Z  RotationAngle=smiData.RigidTransform(28).angle  RotationArbitraryAxis=smiData.RigidTransform(28).axis  FollAlignAxisA=+X  BaseAlignAxisA=+Y  FollAlignAxisB=+Y  BaseAlignAxisB=+Z  RotationSequenceAxes=FollowerAxes  RotationSequence=XYX  RotationSequenceAngles=[0 0 0]  RotationSequenceAnglesUnits=deg  RotationMatrix=[1 0 0; 0 1 0; 0 0 1]
  Transform6 : sm_lib/Frames and Transforms/Rigid Transform  TranslationMethod=Cartesian  TranslationStandardOffset=0  TranslationLengthUnit=mm  TranslationStandardAxis=+Z  TranslationCartesianOffset=smiData.RigidTransform(29).translation  TranslationROffset=0  TranslationROffsetUnits=m  TranslationZOffset=0  TranslationZOffsetUnits=m  TranslationThetaOffset=0  TranslationThetaOffsetUnits=deg  RotationMethod=ArbitraryAxis  RotationAngleUnits=rad  RotationStandardAxis=+Z  RotationAngle=smiData.RigidTransform(29).angle  RotationArbitraryAxis=smiData.RigidTransform(29).axis  FollAlignAxisA=+X  BaseAlignAxisA=+Y  FollAlignAxisB=+Y  BaseAlignAxisB=+Z  RotationSequenceAxes=FollowerAxes  RotationSequence=XYX  RotationSequenceAngles=[0 0 0]  RotationSequenceAnglesUnits=deg  RotationMatrix=[1 0 0; 0 1 0; 0 0 1]
  Transform7 : sm_lib/Frames and Transforms/Rigid Transform  TranslationMethod=Cartesian  TranslationStandardOffset=0  TranslationLengthUnit=mm  TranslationStandardAxis=+Z  TranslationCartesianOffset=smiData.RigidTransform(30).translation  TranslationROffset=0  TranslationROffsetUnits=m  TranslationZOffset=0  TranslationZOffsetUnits=m  TranslationThetaOffset=0  TranslationThetaOffsetUnits=deg  RotationMethod=ArbitraryAxis  RotationAngleUnits=rad  RotationStandardAxis=+Z  RotationAngle=smiData.RigidTransform(30).angle  RotationArbitraryAxis=smiData.RigidTransform(30).axis  FollAlignAxisA=+X  BaseAlignAxisA=+Y  FollAlignAxisB=+Y  BaseAlignAxisB=+Z  RotationSequenceAxes=FollowerAxes  RotationSequence=XYX  RotationSequenceAngles=[0 0 0]  RotationSequenceAnglesUnits=deg  RotationMatrix=[1 0 0; 0 1 0; 0 0 1]
  x03_axe1_RIGID : Subsystem
  x04_manivelle1_RIGID : Subsystem
  x07_roue1_RIGID : Subsystem
  x21_axe1_RIGID : Subsystem
  x22_Rondelle_M03_U1_RIGID : Subsystem
  x24_Anneau_lastique_pour_arbre_008_x_081_RIGID : Subsystem
  F1 : PMIOPort  Side=Right
  F : PMIOPort  Port=2  Side=Right
  F2 : PMIOPort  Port=3  Side=Left
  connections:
  Transform/LConn1 -- ReferenceFrame/RConn1 -- Transform6/LConn1 -- Transform7/LConn1 -- Transform5/LConn1 -- Transform4/LConn1 -- Transform3/LConn1 -- Transform2/LConn1 -- Transform1/LConn1
  Transform/RConn1 -- F/RConn1
  Transform1/RConn1 -- F1/RConn1
  Transform2/RConn1 -- x03_axe1_RIGID/LConn1
  Transform3/RConn1 -- x04_manivelle1_RIGID/LConn1
  Transform4/RConn1 -- x07_roue1_RIGID/LConn1
  Transform5/RConn1 -- x21_axe1_RIGID/LConn1
  Transform6/RConn1 -- x22_Rondelle_M03_U1_RIGID/LConn1
  Transform7/RConn1 -- x24_Anneau_lastique_pour_arbre_008_x_081_RIGID/LConn1
  x07_roue1_RIGID/LConn2 -- F2/RConn1

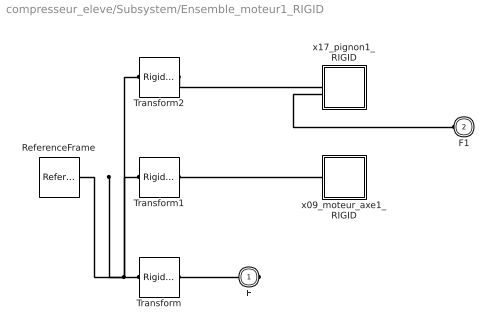
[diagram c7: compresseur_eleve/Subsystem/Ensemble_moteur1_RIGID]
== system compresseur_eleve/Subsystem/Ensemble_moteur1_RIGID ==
  ReferenceFrame : sm_lib/Frames and Transforms/Reference Frame
  Transform : sm_lib/Frames and Transforms/Rigid Transform  TranslationMethod=Cartesian  TranslationStandardOffset=0  TranslationLengthUnit=mm  TranslationStandardAxis=+Z  TranslationCartesianOffset=smiData.RigidTransform(7).translation  TranslationROffset=0  TranslationROffsetUnits=m  TranslationZOffset=0  TranslationZOffsetUnits=m  TranslationThetaOffset=0  TranslationThetaOffsetUnits=deg  RotationMethod=ArbitraryAxis  RotationAngleUnits=rad  RotationStandardAxis=+Z  RotationAngle=smiData.RigidTransform(7).angle  RotationArbitraryAxis=smiData.RigidTransform(7).axis  FollAlignAxisA=+X  BaseAlignAxisA=+Y  FollAlignAxisB=+Y  BaseAlignAxisB=+Z  RotationSequenceAxes=FollowerAxes  RotationSequence=XYX  RotationSequenceAngles=[0 0 0]  RotationSequenceAnglesUnits=deg  RotationMatrix=[1 0 0; 0 1 0; 0 0 1]
  Transform1 : sm_lib/Frames and Transforms/Rigid Transform  TranslationMethod=Cartesian  TranslationStandardOffset=0  TranslationLengthUnit=mm  TranslationStandardAxis=+Z  TranslationCartesianOffset=smiData.RigidTransform(31).translation  TranslationROffset=0  TranslationROffsetUnits=m  TranslationZOffset=0  TranslationZOffsetUnits=m  TranslationThetaOffset=0  TranslationThetaOffsetUnits=deg  RotationMethod=ArbitraryAxis  RotationAngleUnits=rad  RotationStandardAxis=+Z  RotationAngle=smiData.RigidTransform(31).angle  RotationArbitraryAxis=smiData.RigidTransform(31).axis  FollAlignAxisA=+X  BaseAlignAxisA=+Y  FollAlignAxisB=+Y  BaseAlignAxisB=+Z  RotationSequenceAxes=FollowerAxes  RotationSequence=XYX  RotationSequenceAngles=[0 0 0]  RotationSequenceAnglesUnits=deg  RotationMatrix=[1 0 0; 0 1 0; 0 0 1]
  Transform2 : sm_lib/Frames and Transforms/Rigid Transform  TranslationMethod=Cartesian  TranslationStandardOffset=0  TranslationLengthUnit=mm  TranslationStandardAxis=+Z  TranslationCartesianOffset=smiData.RigidTransform(32).translation  TranslationROffset=0  TranslationROffsetUnits=m  TranslationZOffset=0  TranslationZOffsetUnits=m  TranslationThetaOffset=0  TranslationThetaOffsetUnits=deg  RotationMethod=ArbitraryAxis  RotationAngleUnits=rad  RotationStandardAxis=+Z  RotationAngle=smiData.RigidTransform(32).angle  RotationArbitraryAxis=smiData.RigidTransform(32).axis  FollAlignAxisA=+X  BaseAlignAxisA=+Y  FollAlignAxisB=+Y  BaseAlignAxisB=+Z  RotationSequenceAxes=FollowerAxes  RotationSequence=XYX  RotationSequenceAngles=[0 0 0]  RotationSequenceAnglesUnits=deg  RotationMatrix=[1 0 0; 0 1 0; 0 0 1]
  x09_moteur_axe1_RIGID : Subsystem
  x17_pignon1_RIGID : Subsystem
  F : PMIOPort  Side=Right
  F1 : PMIOPort  Port=2  Side=Left
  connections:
  Transform/LConn1 -- ReferenceFrame/RConn1 -- Transform1/LConn1 -- Transform2/LConn1
  Transform/RConn1 -- F/RConn1
  Transform1/RConn1 -- x09_moteur_axe1_RIGID/LConn1
  Transform2/RConn1 -- x17_pignon1_RIGID/LConn1
  F1/RConn1 -- x17_pignon1_RIGID/LConn2
